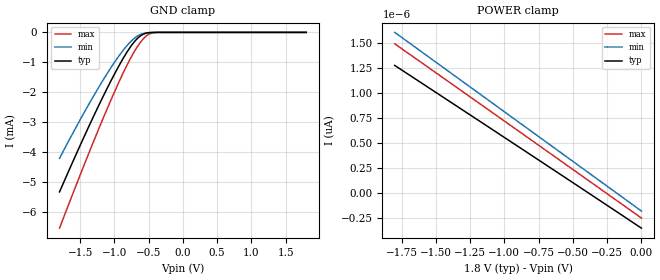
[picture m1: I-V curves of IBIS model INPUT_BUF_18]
| TEXAS INSTRUMENTS INCORPORATED
| Digital Light Processing Group
| IBIS Model of DLP4500FQD
| DLP4500FQD
| This file contains package information for the following:
|  LGA 98-pin S310 package as [Component] DLP4500_S310
| This device can be powered at the following Vccs:
|  2.5 volt Vcc
| This file provides unique models under the [Model Selector] for each Vcc.
| For operation at a specific Vcc, select the appropriate model after each
| [Model Selector] keyword.
[IBIS Ver]   3.2
[Comment char]  |_char
[File Name]   dlpm004.ibs
[File Rev]   2.0 | f_die
[Date]   January 09, 2014
[Source]   Data created from TI-SPICE simulations at TI-DLP.
[Notes]   The following is an IBIS list for the DLP4500FQD.
##notes##|
[Disclaimer] Property of Texas Instruments Incorporated.  Unauthorized
   reproduction and/or distribution is strictly prohibited.
   This product is protected under copyright law.
   Created  2013, (C) Copyright  2013, Texas Instruments
   Incorporated, All Rights Reserved
   UNLESS THERE IS A SIGNED, WRITTEN AGREEMENT TO THE
   CONTRARY, TEXAS INSTRUMENTS (TI) IS PROVIDING THE IBIS
   MODELS  AND WITHOUT ANY WARRANTY, EXPRESSED OR
   IMPLIED.  TI assumes no liability for:
   1) the accuracy of the IBIS models provided to your
   company;
   2) the proper functioning of these IBIS Models in your
   design or for any resulting applications; or
   3) infringement of patents, copyrights or intellectual
   property rights resulting from your use of these IBIS
   models.
   TI provides IBIS Models as a service to our customers.
   You and your company shall not distribute, sell or give
   these models to anyone else without prior written
   permission from TI.
   TI reserves the right to make changes to our products or
   to discontinue any semiconductor product or service
   without notice, and advises our customers to obtain the
   latest version of relevant information to verify, before
   placing orders, that the information being relied on is
   current.
   Please be aware that your receipt and use of the IBIS
   information provided shall serve as acceptance of these
   terms and conditions.  If you do not accept these terms,
   you should return or destroy the IBIS models and any
   other accompanying information immediately.
| Component DLP4500_S310 98-pin LGA
[Component]   DLP4500_S310
[Manufacturer]   Texas Instruments, Inc.
[Package]
|   typ   min   max
R_pkg   5.128E-01   1.176E-01   7.386E-01
L_pkg   3.912E-09   1.712E-09   5.697E-09
C_pkg   1.308E-12   6.679E-13   1.592E-12
[Pin]   signal_name   model_name   R_pin   L_pin   C_pin
A1   DATA(0)   INPUT_BUF   5.279E-01   3.376E-09   1.399E-12
A2   DATA(1)   INPUT_BUF   5.189E-01   3.727E-09   1.469E-12
A3   DATA(2)   INPUT_BUF   5.363E-01   4.382E-09   1.310E-12
A4   DATA(3)   INPUT_BUF   5.489E-01   4.996E-09   1.332E-12
A5   NO_CONNECT NC
A18   NO_CONNECT NC
A19   VOFFSET   POWER
A20   DRC_OEZ   INPUT_BUF   4.900E-01   3.916E-09   1.303E-12
A21   VSS   GND
A22   DRC_STROBE INPUT_BUF   5.031E-01   3.469E-09   1.323E-12
B1   DATA(4)   INPUT_BUF   5.536E-01   3.850E-09   1.353E-12
B2   VSS   GND
B3   DATA(5)   INPUT_BUF   5.398E-01   4.234E-09   1.364E-12
B4   VSS   GND
B5   NO_CONNECT NC
B18   NO_CONNECT NC
B19   VREF   POWER
B20   VSS   GND
B21   DRC_BUS   INPUT_BUF   4.823E-01   3.623E-09   1.337E-12
B22   VCC   POWER
C1   DATA(6)   INPUT_BUF   5.396E-01   3.510E-09   1.375E-12
C2   VCC   POWER
C3   DATA(7)   INPUT_BUF   5.437E-01   4.276E-09   1.232E-12
C4   DATA(8)   INPUT_BUF   5.444E-01   4.671E-09   1.394E-12
C5   NO_CONNECT NC
C18   NO_CONNECT NC
C19   VBIAS   POWER
C20   SAC_BUS   INPUT_BUF   4.858E-01   3.746E-09   1.493E-12
C21   VSS   GND
C22   SAC_CLK   INPUT_BUF   2.222E-01   2.293E-09   8.613E-13
D1   DATA(9)   INPUT_BUF   5.271E-01   3.200E-09   1.289E-12
D2   VSS   GND
D3   VSS   GND
D4   DATA(10)   INPUT_BUF   5.407E-01   4.588E-09   1.421E-12
D5   NO_CONNECT NC
D18   NO_CONNECT NC
D19   VBIAS   POWER
D20   VSS   GND
D21   VCC   POWER
D22   VSS   GND
E1   DATA(11)   INPUT_BUF   5.308E-01   3.721E-09   1.412E-12
E2   VCC   POWER
E3   VSS   GND
E4   DATA(12)   INPUT_BUF   5.448E-01   4.808E-09   1.275E-12
E5   NO_CONNECT NC
E18   NO_CONNECT NC
E19   VRESET   POWER
E20   VCC   POWER
E21   VSS   GND
E22   VCC   POWER
F1   DATA(13)   INPUT_BUF   5.342E-01   3.584E-09   1.255E-12
F2   VSS   GND
F3   DATA(14)   INPUT_BUF   5.276E-01   3.961E-09   1.247E-12
F4   VSS   GND
F5   NO_CONNECT NC
F18   NO_CONNECT NC
F19   VRESET   POWER
F20   VSS   GND
F21   VCC   POWER
F22   VSS   GND
G1   DATA(15)   INPUT_BUF   5.249E-01   3.257E-09   1.202E-12
G2   DATA(16)   INPUT_BUF   5.423E-01   3.875E-09   1.342E-12
G3   VCC   POWER
G4   DATA(17)   INPUT_BUF   5.340E-01   4.545E-09   1.592E-12
G5   NO_CONNECT NC
G18   NO_CONNECT NC
G19   VCC   POWER
G20   VCC   POWER
G21   VSS   GND
G22   VCC   POWER
H1   DATA(18)   INPUT_BUF   5.310E-01   3.284E-09   1.243E-12
H2   DATA(19)   INPUT_BUF   5.229E-01   3.659E-09   1.319E-12
H3   VSS   GND
H4   DATA(20)   INPUT_BUF   5.328E-01   4.412E-09   1.434E-12
H5   NO_CONNECT NC
H18   NO_CONNECT NC
H19   VCC   POWER
H20   VSS   GND
H21   VCC   POWER
H22   VSS   GND
J1   DATA(21)   INPUT_BUF   5.346E-01   3.670E-09   1.275E-12
J2   VSS   GND
J3   DATA(22)   INPUT_BUF   5.316E-01   3.932E-09   1.335E-12
J4   DATA(23)   INPUT_BUF   5.381E-01   4.430E-09   1.334E-12
J5   NO_CONNECT NC
J18   NO_CONNECT NC
J19   VREF   POWER
J20   VCC   POWER
J21   VSS   GND
J22   VCC   POWER
K1   DCLK   INPUT_BUF   5.460E-01   3.785E-09   1.301E-12
K2   LOADB   INPUT_BUF   5.080E-01   4.141E-09   1.319E-12
K3   SCTRL   INPUT_BUF   5.126E-01   3.944E-09   1.363E-12
K4   TRC   INPUT_BUF   7.386E-01   5.697E-09   1.570E-12
K19   VOFFSET   POWER
K20   VSS   GND
K21   VCC   POWER
K22   NO_CONNECT NC
| Model INPUT_BUF
[Model Selector]   INPUT_BUF
INPUT_BUF_18   1.8 volt Vcc
| Models and submodels in the file (1): INPUT_BUF_18 (Input)
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[Model]   INPUT_BUF_18
Model_type  Input
Vinl=0.36
Vinh=1.44
| variable   typ   min   max
C_comp   0.29pF   0.23pF   0.31pF
[Temperature Range]   40   100   0
| Ambient temperature   25   85   -40
[Voltage range]   1.8   1.65   1.95
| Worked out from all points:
|   GND clamp passes 1 mA (typ) near -0.90 V on its own axis
[GND Clamp]
| INPUT_BUF_18
|   Voltage   I(typ)   I(min)   I(max)
-1.8V     -5.319mA   -4.198mA   -6.527mA
-1.545V   -4.001mA   -3.106mA   -5.023mA
-1.32V    -2.88mA    -2.189mA   -3.733mA
-1.12V    -1.934mA   -1.427mA   -2.63mA
-950mV    -1.186mA   -840.2uA   -1.741mA
-820mV    -673.5uA   -453.5uA   -1.113mA
-715mV    -332.5uA   -209.4uA   -667.5uA
-625mV    -127.6uA   -75.21uA   -349uA
-535mV    -27.06uA   -17.14uA   -121.4uA
-460mV    -4.641uA   -3.582uA   -29.58uA
-355mV    -235.9nA   -285.7nA   -1.811uA
1.8V      14.91pA    62.54pA    31.07pA
[POWER Clamp]
| INPUT_BUF_18
|   Voltage   I(typ)   I(min)   I(max)
-1.8V     1.275pA    1.605pA    1.491pA
-830mV    403.9fA    644.9fA    556.4fA
-405mV    19.82fA    224fA      145.4fA
-16.28fV  -347.9fA   -177.3fA   -247.1fA
